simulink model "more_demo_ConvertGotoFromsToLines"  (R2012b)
settings: Solver=ode45  SolverMode=SingleTasking  StartTime=0.0  StopTime=10.0  RelTol=1e-3

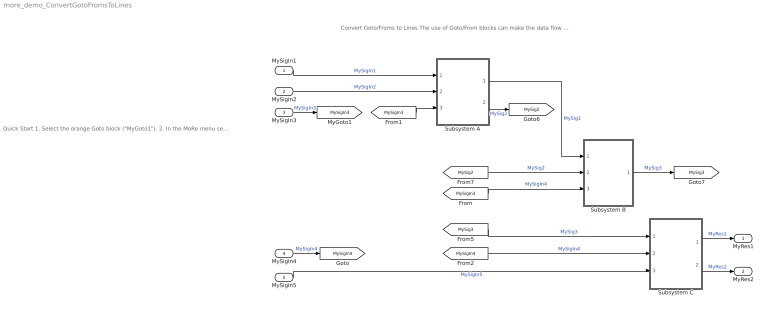
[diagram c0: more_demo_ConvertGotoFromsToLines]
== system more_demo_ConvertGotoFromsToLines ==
  note: Quick Start 1. Select the orange Goto block ("MyGoto1"). 2. In the MoRe menu select "Signal Routing-> Convert Goto/Froms to Lines" and note the changes. 3. Now deselect all blocks, apply the action again and note the changes.
  note: Convert Goto/Froms to Lines The use of Goto/From blocks can make the data flow in the model difficult to follow. With this action you can convert Goto/From blocks to lines to make the data flow clearer.
  MySigIn1 : Inport
  MySigIn2 : Inport  Port=2
  MySigIn3 : Inport  Port=3
  MySigIn4 : Inport  Port=4
  MySigIn5 : Inport  Port=5
  Subsystem A : Subsystem
  Subsystem B : Subsystem
  Subsystem C : Subsystem
  MyRes1 : Outport
  MyRes2 : Outport  Port=2
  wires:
  MySigIn1/1 -> Subsystem A/1(MySigIn1)  "MySigIn1"
  MySigIn2/1 -> Subsystem A/2(MysigIn2)  "MySigIn2"
  Subsystem A/1(MySig1) -> Subsystem B/1(MySig1)  "MySig1"
  Subsystem C/1(MyRes1) -> MyRes1/1  "MyRes1"
  Subsystem C/2(MyRes2) -> MyRes2/1  "MyRes2"
  MySigIn5/1 -> Subsystem C/3(MySigIn5)  "MySigIn5"
  [MySig3] -> Subsystem C/1(MySig3)  "MySig3"
  Subsystem B/1(MySig3) -> [MySig3]  "MySig3"
  [MySig2] -> Subsystem B/2(MySig2)  "MySig2"
  Subsystem A/2(MySig2) -> [MySig2]  "MySig2"
  [MySigIn3] -> Subsystem B/3(MySigIn4)  "MySigIn4"
  [MySigIn3] -> Subsystem A/3(MySigIn3)
  MySigIn3/1 -> [MySigIn3]  "MySigIn3"
  [MySigIn4] -> Subsystem C/2(MySigIn4)  "MySigIn4"
  MySigIn4/1 -> [MySigIn4]  "MySigIn4"

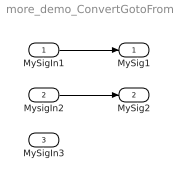
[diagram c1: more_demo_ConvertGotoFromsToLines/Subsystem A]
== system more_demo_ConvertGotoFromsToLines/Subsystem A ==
  MySigIn1 : Inport
  MysigIn2 : Inport  Port=2
  MySigIn3 : Inport  Port=3
  MySig1 : Outport
  MySig2 : Outport  Port=2
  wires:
  MySigIn1/1 -> MySig1/1
  MysigIn2/1 -> MySig2/1
  MySigIn3/1 -> ?

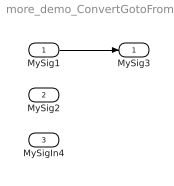
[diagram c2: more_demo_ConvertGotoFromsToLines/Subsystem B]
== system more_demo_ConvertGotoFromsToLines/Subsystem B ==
  MySig1 : Inport
  MySig2 : Inport  Port=2
  MySigIn4 : Inport  Port=3
  MySig3 : Outport
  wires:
  MySig1/1 -> MySig3/1

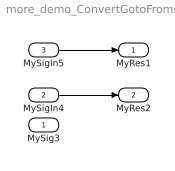
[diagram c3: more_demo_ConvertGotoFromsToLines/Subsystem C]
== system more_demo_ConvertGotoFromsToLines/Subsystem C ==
  MySig3 : Inport
  MySigIn4 : Inport  Port=2
  MySigIn5 : Inport  Port=3
  MyRes1 : Outport
  MyRes2 : Outport  Port=2
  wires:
  MySigIn5/1 -> MyRes1/1
  MySigIn4/1 -> MyRes2/1
